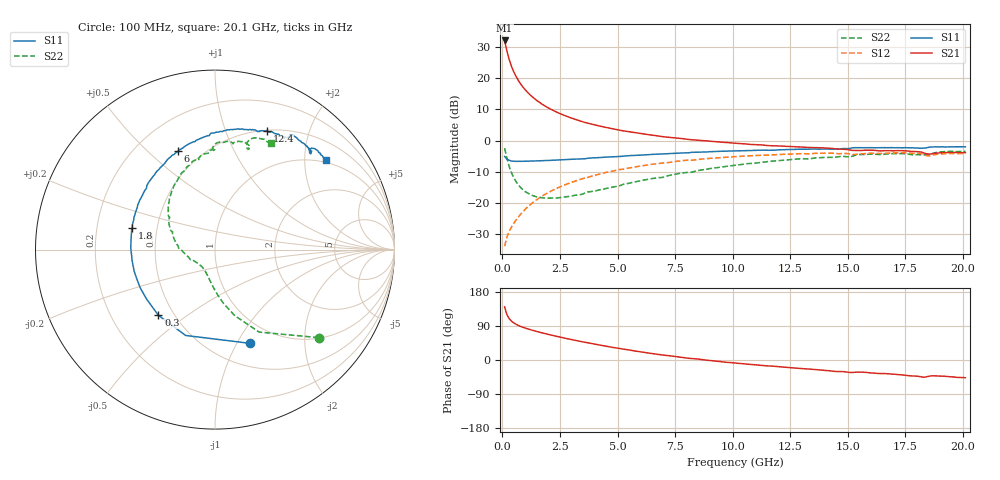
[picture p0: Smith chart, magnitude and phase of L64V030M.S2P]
!  Infineon Technologies AG
! BFR380L3 , PF131585-7, No.6, Th 09.10.01, soldered on pcb-board, measured with PP GSG850
!  Vce=4.0 V,  Ic=30.0 mA
! Common Emitter S-Parameters:  15. November 2001
#  GHz  S  MA  R  50
! f  S11  S21  S12  S22
! GHz  Mag  Ang  Mag  Ang  Mag  Ang  Mag  Ang
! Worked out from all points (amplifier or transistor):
!   201 points, 100 MHz to 20.1 GHz, reference 50 ohm
!   highest |S21| = 32.1 dB at 100 MHz (marker M1)
!   |S21| within 3 dB of that: start of sweep to 188.9 MHz
!   unconditionally stable (mu >= 1): 1.245 GHz to 4.344 GHz
!   at 3.4 GHz: K = 1.02, MAG = 8.5 dB, |S12| = -12.4 dB
!   at 10.1 GHz: K = 0.95, MSG = 2.1 dB, |S12| = -5.2 dB
!   at 20.1 GHz: K = 0.98, MSG = 0.1 dB, |S12| = -4.1 dB
!   S11 on the Smith chart (normalised r, x): 100 MHz: 0.75, -1.13; 300 MHz: 0.41, -0.39; 1.8 GHz: 0.36, +0.11; 6 GHz: 0.37, +0.63; 12.4 GHz: 0.51, +1.40; 20.1 GHz: 0.94, +2.52
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0.1  0.5572 -69.6  40.08 140.3  0.02042 65.5  0.7575 -40.4
0.2  0.5055 -108.9  27.18 119.6  0.02845 56.5  0.5213 -61.8
0.3  0.4831 -130.8  19.79 109.1  0.03552 56.8  0.3846 -73.3
0.4  0.4704 -144.1  15.39 102.4  0.04125 58.1  0.3045 -80.9
0.5  0.468 -153.0  12.53 97.8  0.04742 60.3  0.2535 -86.6
0.6  0.4651 -159.7  10.56 94.2  0.0538 61.9  0.2192 -91.2
0.7  0.4662 -164.9  9.124 91.2  0.05984 63.1  0.1943 -95.3
0.8  0.4652 -169.3  8.029 88.5  0.06665 64.3  0.1762 -98.9
1  0.4656 -176.2  6.474 84.2  0.07989 65.5  0.1521 -105.3
1.2  0.4694 178.0  5.428 80.3  0.09337 66.1  0.1378 -111.1
1.5  0.4727 171.1  4.38 75.1  0.1137 66.1  0.1256 -118.8
1.8  0.4774 165.2  3.679 70.5  0.1343 65.3  0.1205 -125.9
2.5  0.4906 153.2  2.707 60.5  0.1813 62.2  0.1223 -140.3
3.5  0.5117 138.8  1.997 47.7  0.2471 56.3  0.1394 -156.2
4.6  0.5449 125.1  1.594 35.3  0.315 49.2  0.1742 -173.8
6  0.5862 110.5  1.299 21.5  0.3913 39.7  0.2276 168.0
6.8  0.6091 102.8  1.18 14.5  0.4317 33.9  0.2556 158.0
10.1  0.6845 78.4  0.9062 -7.9  0.5526 12.3  0.4034 126.8
12.4  0.7204 66.4  0.8078 -19.6  0.608 -1.8  0.4915 107.2
13.5  0.7307 61.2  0.7733 -24.7  0.6208 -8.3  0.5213 99.5
16.8  0.7693 48.6  0.6897 -36.5  0.6294 -24.4  0.6143 78.5
20.1  0.7925 38.9  0.643 -46.7  0.6241 -38.1  0.6734 62.3
